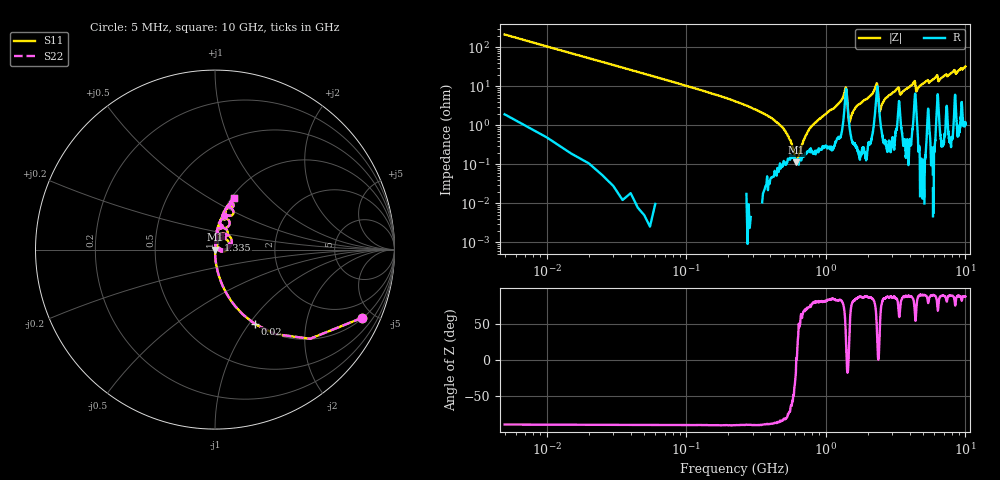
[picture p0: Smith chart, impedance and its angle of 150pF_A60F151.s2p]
! Amotech Co.,Ltd.
! http://www.amotech.co.kr/
! Part Number: A60F151
! These Parameters are Measured in Series Mode Connection
! Operation Temp=25[degC], DC Bias Voltage=0[V]
! Freq. Start=5[MHz] Stop=10[GHz], 2000[Steps]
! Date: Monday, July 20, 2020, 03:46:34
# GHZ S RI R 50.000000
!Freq.(Hz) S11(Real) S11(Imag) S21(Real) S21(Imag) S12(Real) S12(Imag) S22(Real) S22(Imag)
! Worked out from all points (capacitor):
!   2000 points, 5 MHz to 10 GHz, reference 50 ohm
!   read as one part in series: C = 149 pF near 55 MHz
!   lowest |Z| = 112 mohm at 615 MHz (marker M1)
!   series resonance near 614.5 MHz, so ESL is about 450 pH
!   S11 on the Smith chart (normalised r, x): 5 MHz: 1.04, -4.30; 20 MHz: 1.00, -1.06; 1.335 GHz: 1.03, +0.11; 10 GHz: 1.02, +0.65
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0.005  0.8198 -0.3799  0.1802 0.3799  0.1802 0.3799  0.8198 -0.3799
0.02  0.2212 -0.4141  0.7788 0.4141  0.7788 0.4141  0.2212 -0.4141
0.09  0.0131 -0.1142  0.9869 0.1142  0.9869 0.1142  0.0131 -0.1142
0.465  0.000969 -0.0104  0.999 0.0104  0.999 0.0104  0.000969 -0.0104
0.615  0.00112 5.17e-05  0.9989 -5.17e-05  0.9989 -5.17e-05  0.00112 5.17e-05
0.815  0.00197 0.0102  0.998 -0.0102  0.998 -0.0102  0.00197 0.0102
1.335  0.0156 0.0522  0.9844 -0.0522  0.9844 -0.0522  0.0156 0.0522
1.39  0.0741 0.046  0.9259 -0.046  0.9259 -0.046  0.0741 0.046
1.495  0.00693 0.0117  0.9931 -0.0117  0.9931 -0.0117  0.00693 0.0117
1.675  0.00366 0.0318  0.9963 -0.0318  0.9963 -0.0318  0.00366 0.0318
2.295  0.0564 0.088  0.9436 -0.088  0.9436 -0.088  0.0564 0.088
2.45  0.0141 0.0185  0.9859 -0.0185  0.9859 -0.0185  0.0141 0.0185
2.69  0.00626 0.0499  0.9937 -0.0499  0.9937 -0.0499  0.00626 0.0499
3.34  0.0456 0.0726  0.9544 -0.0726  0.9544 -0.0726  0.0456 0.0726
3.44  0.015 0.0595  0.985 -0.0595  0.985 -0.0595  0.015 0.0595
4.3  0.0458 0.1211  0.9542 -0.1211  0.9542 -0.1211  0.0458 0.1211
4.465  0.0247 0.0689  0.9753 -0.0689  0.9753 -0.0689  0.0247 0.0689
5.005  0.0152 0.1184  0.9848 -0.1184  0.9848 -0.1184  0.0152 0.1184
6.67  0.0294 0.1553  0.9706 -0.1553  0.9706 -0.1553  0.0294 0.1553
8.335  0.0869 0.2336  0.9131 -0.2336  0.9131 -0.2336  0.0869 0.2336
8.545  0.0664 0.1924  0.9336 -0.1924  0.9336 -0.1924  0.0664 0.1924
10  0.1034 0.2868  0.8966 -0.2868  0.8966 -0.2868  0.1034 0.2868
